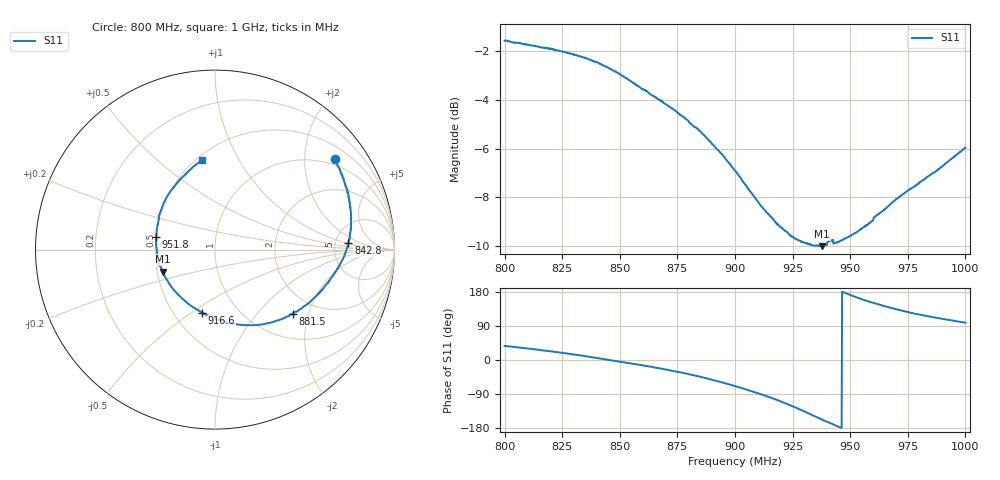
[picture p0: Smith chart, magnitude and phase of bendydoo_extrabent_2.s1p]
# HZ S RI R 50
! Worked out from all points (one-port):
!   1010 points, 800 MHz to 1 GHz, reference 50 ohm
!   lowest |S11| = -10.0 dB at 937.8 MHz (marker M1), VSWR 1.92, Z = 26.8 - j7.26 ohm
!   |S11| at or under -10 dB: 935.1029 MHz to 935.321 MHz (218.1 kHz wide, 0.0233 % of centre); 936.1639 MHz to 936.4721 MHz (308.2 kHz wide, 0.0329 % of centre); 937.6066 MHz to 937.9713 MHz (364.7 kHz wide, 0.0389 % of centre)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
!   S11 on the Smith chart (normalised r, x): 800 MHz: 0.83, +2.76; 842.8 MHz: 6.64, +1.05; 881.5 MHz: 1.53, -1.59; 916.6 MHz: 0.68, -0.55; 951.8 MHz: 0.50, +0.08; 1 GHz: 0.53, +0.71
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8e8  0.6672 0.5037
8.124876e8  0.7148 0.3931
8.251734e8  0.7507 0.2562
8.352824e8  0.7585 0.1321
8.428147e8  0.7431 0.0353
8.501486e8  0.7096 -0.0575
8.616452e8  0.6335 -0.1793
8.685827e8  0.5724 -0.2489
8.751239e8  0.5076 -0.3083
8.814668e8  0.4319 -0.3565
8.846382e8  0.3937 -0.3762
8.907829e8  0.3024 -0.4087
8.949455e8  0.2411 -0.4193
9.000991e8  0.1624 -0.4203
9.080277e8  0.0416 -0.3987
9.16551e8  -0.0724 -0.3505
9.250743e8  -0.1765 -0.2789
9.318136e8  -0.2461 -0.2023
9.377601e8  -0.291 -0.122
9.415262e8  -0.316 -0.0734
9.437066e8  -0.3182 -0.0394
9.500495e8  -0.3277 0.0488
9.518335e8  -0.3274 0.0724
9.617443e8  -0.3095 0.1955
9.692765e8  -0.2772 0.2761
9.750247e8  -0.245 0.3294
9.849355e8  -0.1805 0.4044
9.999999e8  -0.0727 0.4979
